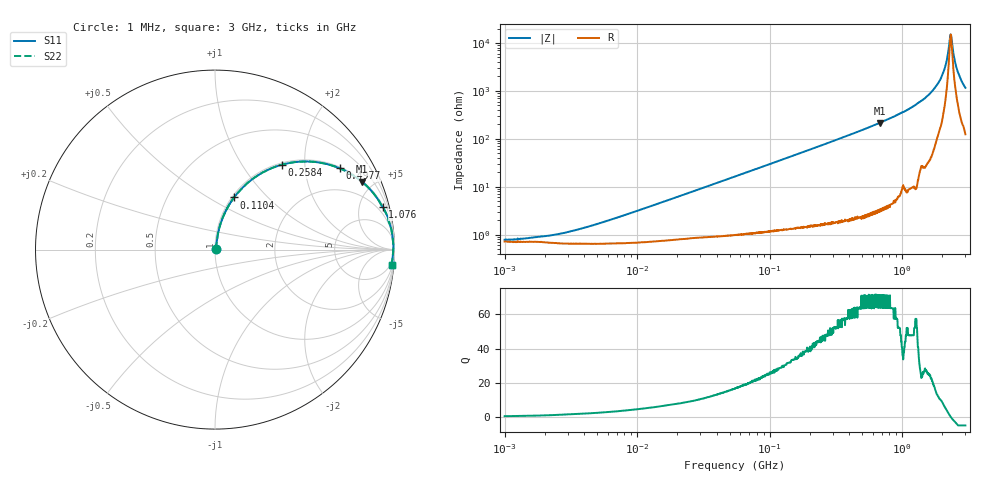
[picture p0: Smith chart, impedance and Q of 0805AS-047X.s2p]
!s-Parameter Generated by FASTRON Sdn. Bhd.
!FASTRON P/N : 0805AS-047X
!Keysight Technologies: E4991B_MY54100416_A.01.15
!Date: Mon Jun 15 12:50:37 2026
!Version  :Rev01  Mon Jun 15 12:50:37 2026
!Data & Calibration Information:
!Freq  S11  S21  S12  S22
!PortZ  Port1:50+j0  Port2:50+j0
!When reading reference impedance value at option line is always used.
! Remarks : This data is being provided solely for informational purposes.
# Hz S dB R 50
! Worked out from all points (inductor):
!   1601 points, 1 MHz to 3 GHz, reference 50 ohm
!   read as one part in series: L = 48.8 nH near 6.369 MHz
!   highest Q = 71.2 at 675.3 MHz (marker M1), where L = 50.5 nH
!   self-resonance near 2.324 GHz
!   S11 on the Smith chart (normalised r, x): 1 MHz: 1.01, +0.01; 110.4 MHz: 1.02, +0.66; 258.4 MHz: 1.03, +1.53; 497.7 MHz: 1.04, +3.04; 1.076 GHz: 1.16, +7.80; 3 GHz: 3, -23
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1000000  -42.20 23.1  -0.06 -0.2  -0.06 -0.2  -42.20 23.1
2150303  -40.50 44.1  -0.06 -0.4  -0.06 -0.4  -40.50 44.1
3804036  -37.50 60.5  -0.06 -0.7  -0.06 -0.7  -37.50 60.5
1.447069e7  -27.10 78.1  -0.07 -2.5  -0.07 -2.5  -27.10 78.1
5.504702e7  -15.90 77.3  -0.20 -9.2  -0.20 -9.2  -15.90 77.3
1.103592e8  -10.20 70.0  -0.54 -17.9  -0.54 -17.9  -10.20 70.0
2.083556e8  -5.69 57.3  -1.49 -31.3  -1.49 -31.3  -5.69 57.3
2.583764e8  -4.40 51.7  -2.10 -37.0  -2.10 -37.0  -4.40 51.7
4.976708e8  -1.62 33.1  -5.26 -56.0  -5.26 -56.0  -1.62 33.1
6.753166e8  -0.91 24.9  -7.52 -64.3  -7.52 -64.3  -0.91 24.9
7.925923e8  -0.64 20.9  -8.94 -68.2  -8.94 -68.2  -0.64 20.9
1.075512e9  -0.32 14.3  -12.20 -74.5  -12.20 -74.5  -0.32 14.3
1.526649e9  -0.12 7.5  -17.70 -80.3  -17.70 -80.3  -0.12 7.5
1.855641e9  -0.07 4.0  -23.10 -81.4  -23.10 -81.4  -0.07 4.0
2.071593e9  -0.06 2.1  -28.60 -79.1  -28.60 -79.1  -0.06 2.1
2.156205e9  -0.05 1.4  -32.10 -75.0  -32.10 -75.0  -0.05 1.4
2.266846e9  -0.05 0.5  -39.70 -52.7  -39.70 -52.7  -0.05 0.5
2.324278e9  -0.06 0.0  -43.60 -2.8  -43.60 -2.8  -0.06 0.0
2.383164e9  -0.06 -0.4  -39.70 46.9  -39.70 46.9  -0.06 -0.4
2.51802e9  -0.07 -1.4  -31.70 70.7  -31.70 70.7  -0.07 -1.4
2.634014e9  -0.08 -2.2  -27.90 76.1  -27.90 76.1  -0.08 -2.2
3e9  -0.11 -4.8  -21.40 79.0  -21.40 79.0  -0.11 -4.8
